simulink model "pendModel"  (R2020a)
settings: Solver=VariableStepAuto  StartTime=0.0  StopTime=10.0  RelTol=1e-3
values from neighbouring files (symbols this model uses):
  b = 1    [initParams.m]
  g = 9.81    [initParams.m]
  m = 0.5    [initParams.m]
  R = 0.7    [initParams.m]
  x0 = [0.2;0.1]    [initParams.m]

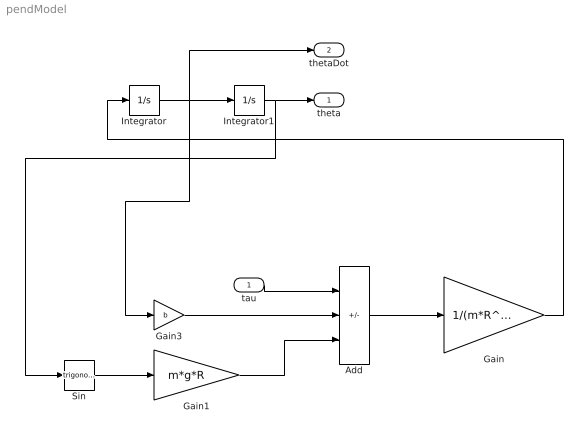
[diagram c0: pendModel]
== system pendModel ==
  tau : Inport
  Add : Sum  Inputs=+--
  Gain : Gain  Gain=1/(m*R^2)
  Gain1 : Gain  Gain=m*g*R
  Gain3 : Gain  Gain=b
  Integrator : Integrator  InitialCondition=x0(1)
  Integrator1 : Integrator  InitialCondition=x0(2)
  Sin : Trigonometry
  theta : Outport
  thetaDot : Outport  Port=2
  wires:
  Integrator/1 -> Gain3/1, thetaDot/1, Integrator1/1
  Integrator1/1 -> Sin/1, theta/1
  tau/1 -> Add/1
  Gain3/1 -> Add/2
  Sin/1 -> Gain1/1
  Gain1/1 -> Add/3
  Add/1 -> Gain/1
  Gain/1 -> Integrator/1
